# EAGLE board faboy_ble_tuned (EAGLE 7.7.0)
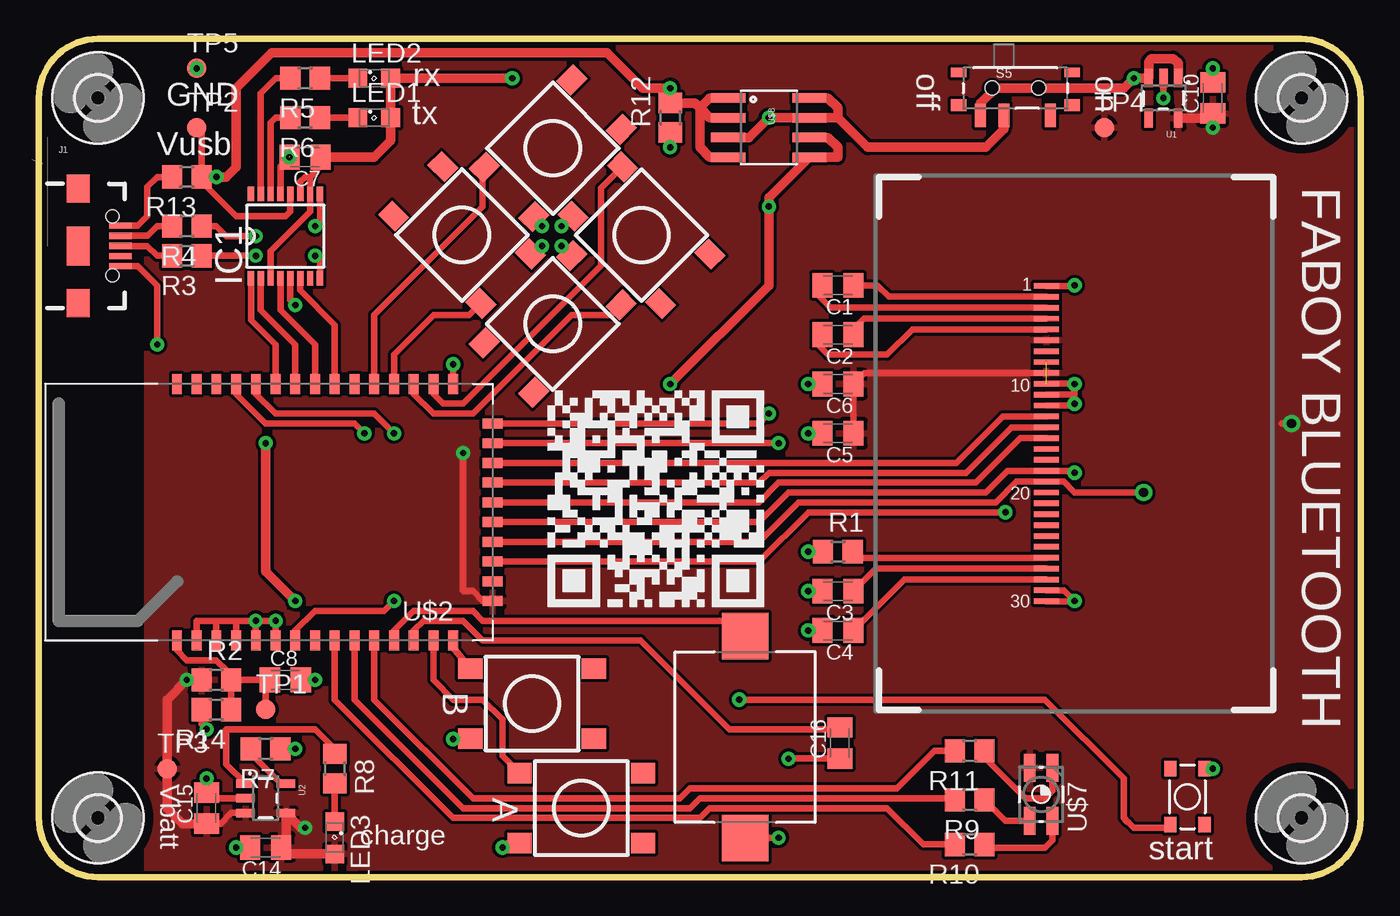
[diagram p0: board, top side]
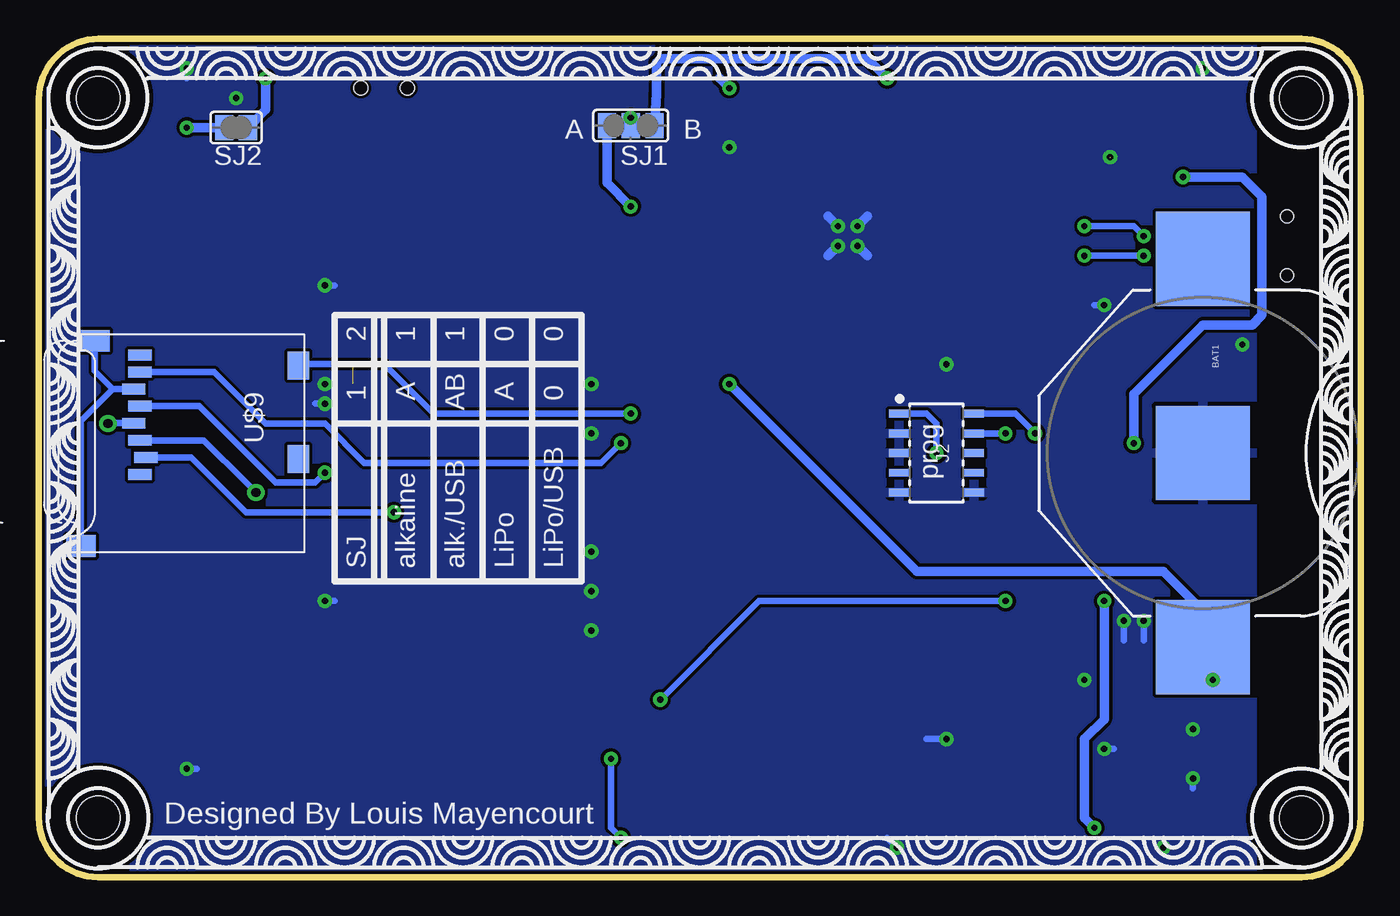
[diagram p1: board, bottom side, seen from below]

Size 85.09 x 53.98 mm. Coordinates in mm from the lower left corner, seen from the top.
Outline: 81.23,53.98 3.81,53.98 arc90 0,50.16 0,3.81 arc90 3.81,0 81.28,0 arc90 85.09,3.81 85.09,50.11 arc90 81.23,53.98
Copper layers (1*16): Top 0.035mm / dielectric 1.5mm / Bottom 0.035mm
Design rules "SparkFun": minimum track width 8mil, minimum drill 20mil, track to track 8mil, track to pad 8mil, pad to pad 8mil, via to via 8mil, smd to smd 8mil, copper to edge 8mil, drill to drill 8mil, minimum pad ring 12mil, minimum via ring 10mil, stop-mask expansion 4mil, vias tented up to drill 20mil, thermal gap 10mil

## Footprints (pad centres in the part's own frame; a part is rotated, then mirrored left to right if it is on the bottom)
BATTCON_20MM = smd 6.07 x 6.07: 1 -12.5,0; 2 0,0; 3 12.5,0
C0805K = smd 1.3 x 1.6: 1 -1,0; 2 1,0
SSOP16 = smd 0.914 x 0.406: 1 -2.718,2.223; 2 -2.718,1.587; 3 -2.718,0.953; 4 -2.718,0.318; 5 -2.718,-0.318; 6 -2.718,-0.953; 7 -2.718,-1.587; 8 -2.718,-2.223; 9 2.718,-2.223; 10 2.718,-1.587; 11 2.718,-0.953; 12 2.718,-0.318; 13 2.718,0.318; 14 2.718,0.953; 15 2.718,1.587; 16 2.718,2.223
USB-B-MICRO-SMD_V03_RED_PASTE = smd 1.45 x 0.4: D+ 2.725,0; D- 2.725,0.65; GND 2.725,-1.3; ID 2.725,-0.65; VBUS 2.725,1.3 | smd 1.5 x 1.8: SHIELD1 0,3.685; SHIELD2 0,-3.685 | smd 1.5 x 2.5: SHIELD3 0,0 | hole 0.85: 2.2,1.9; 2.2,-1.9
SAMTECH_FTSH-105-01 = smd 0.508 x 1.27: 1 -2.54,-2.413; 2 -2.54,2.413; 3 -1.27,-2.413; 4 -1.27,2.413; 5 0,-2.413; 6 0,2.413; 7 1.27,-2.413; 8 1.27,2.413; 9 2.54,-2.413; 10 2.54,2.413
SML0805 = smd 1.2 x 1.2: A 1.05,0; C -1.05,0
R0805 = smd 1.3 x 1.5: 1 -0.95,0; 2 0.95,0
TACTILE_SWITCH_TALL = smd 1.55 x 1.3: A1 -3.975,-2.25; A2 3.975,-2.25; B1 -3.975,2.25; B2 3.975,2.25
SWITCH-SPST-SMD-A = smd 0.7 x 1.5: 1 -2.25,-1.75; 2 -0.75,-1.75; 3 2.25,-1.75 | smd 1 x 0.6: GND1 -3.65,1; GND3 3.65,1 | smd 1 x 0.8: GND2 -3.65,-1.1; GND4 3.65,-1.1 | hole 0.9: -1.5,0; 1.5,0
TACTILE_SWITCH_SMD-3 = smd 1 x 0.8: 1 -1.8,1.1; 2 1.8,1.1; 3 -1.8,-1.1; 4 1.8,-1.1
BUZZER-CMT1102 = smd 3 x 3: 1 -6.5,0; 2 6.5,0
SJ_2 = smd 1.168 x 1.6: 1 -1.524,0; 2 0,0; 3 1.524,0
SJ = smd 1.168 x 1.6: 1 -0.762,0; 2 0.762,0
B1,27 = smd 1.27 x 1.27: TP 0,0
SOT23-5 = smd 0.55 x 1.2: 1 -0.95,-1.3; 2 0,-1.3; 3 0.95,-1.3; 4 0.95,1.3; 5 -0.95,1.3
1X30-0.7MM = smd 0.35 x 1.6: 1 -10.15,0; 2 -9.45,0; 3 -8.75,0; 4 -8.05,0; 5 -7.35,0; 6 -6.65,0; 7 -5.95,0; 8 -5.25,0; 9 -4.55,0; 10 -3.85,0; 11 -3.15,0; 12 -2.45,0; 13 -1.75,0; 14 -1.05,0; 15 -0.35,0; 16 0.35,0; 17 1.05,0; 18 1.75,0; 19 2.45,0; 20 3.15,0; 21 3.85,0; 22 4.55,0; 23 5.25,0; 24 5.95,0; 25 6.65,0; 26 7.35,0; 27 8.05,0; 28 8.75,0; 29 9.45,0; 30 10.15,0
WT51822 = smd 1.27 x 0.635: 1 0,13.97; 2 0,12.7; 3 0,11.43; 4 0,10.16; 5 0,8.89; 6 0,7.62; 7 0,6.35; 8 0,5.08; 9 0,3.81; 10 0,2.54 | smd 0.635 x 1.27: 11 2.54,0; 12 3.81,0; 13 5.08,0; 14 6.35,0; 15 7.62,0; 16 8.89,0; 17 10.16,0; 18 11.43,0; 19 12.7,0; 20 13.97,0; 21 15.24,0; 22 16.51,0; 23 17.78,0; 24 19.05,0; 25 20.32,0; 26 20.32,16.51; 27 19.05,16.51; 28 17.78,16.51; 29 16.51,16.51; 30 15.24,16.51; 31 13.97,16.51; 32 12.7,16.51; 33 11.43,16.51; 34 10.16,16.51; 35 8.89,16.51; 36 7.62,16.51; 37 6.35,16.51; 38 5.08,16.51; 39 3.81,16.51; 40 2.54,16.51
2,8 = hole 2.8: 0,0
P-LCC-4-3 = smd 0.75 x 1.8: 1 0.725,1.7; 2 -0.725,1.7; 3 -0.725,-1.7; 4 0.725,-1.7
SO08 = smd 0.61 x 2.21: 1 -1.905,-2.616; 2 -0.635,-2.616; 3 0.635,-2.616; 4 1.905,-2.616; 5 1.905,2.616; 6 0.635,2.616; 7 -0.635,2.616; 8 -1.905,2.616
MICROSD = smd 0.7 x 1.5: 1 9,-10.64; 2 7.9,-10.24; 3 6.8,-10.64; 4 5.7,-11.04; 5 4.6,-10.64; 6 3.5,-11.04; 7 2.4,-10.64; 8 1.3,-10.64 | smd 1.8 x 1.4: CD1 2,-0.44; CD2 8,-0.44 | smd 1.4 x 1.9: MT1 0.4,-13.54; MT2 13.6,-14.44

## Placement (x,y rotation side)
BAT1  [BATTCON_20MM]  10.16,27.3 270 bottom
C1  1uF  [C0805K]  51.44,38.1 180 top
C2  1uF  [C0805K]  51.44,34.92 180 top
C3  4.7uF / 10v  [C0805K]  51.44,18.41 180 top
C4  2.2uF  [C0805K]  51.44,15.88 180 top
C5  1uF  [C0805K]  51.44,28.57 180 top
C6  1uF  [C0805K]  51.44,31.75 180 top
C7  0.1uF  [C0805K]  17.14,46.35 180 top
C8  22nF  [C0805K]  15.88,12.7 0 top
C10  2.2uF  [C0805K]  75.56,50.16 90 top
C14  4.7uF  [C0805K]  14.61,1.91 180 top
C15  4.7uF  [C0805K]  10.79,4.45 90 top
C16  4.7uF  [C0805K]  51.56,8.64 90 top
IC1  FT230XS  [SSOP16]  15.88,41.27 90 top
J1  USB-MICROBREDUCED_PASTE  [USB-B-MICRO-SMD_V03_RED_PASTE]  2.54,40.64 0 top
J2  CORTEX_DEBUGSMD  [SAMTECH_FTSH-105-01]  27.3,27.3 270 bottom
LED1  [SML0805]  21.59,48.9 0 top
LED2  [SML0805]  21.59,51.44 0 top
LED3  [SML0805]  19.05,2.54 270 top
R1  390k  [R0805]  51.44,20.95 0 top
R2  10M  [R0805]  11.43,12.7 0 top
R3  22  [R0805]  9.53,40.01 180 top
R4  22  [R0805]  9.53,41.91 180 top
R5  820  [R0805]  17.14,51.44 180 top
R6  820  [R0805]  17.14,48.9 180 top
R7  390k  [R0805]  14.61,8.26 180 top
R8  470  [R0805]  19.05,6.99 270 top
R9  820  [R0805]  59.92,4.98 180 top
R10  820  [R0805]  59.92,2.11 180 top
R11  820  [R0805]  59.92,8.13 180 top
R12  10k  [R0805]  40.64,48.9 90 top
R13  ferrite  [R0805]  9.53,45.09 180 top
R14  2.2M  [R0805]  11.43,10.79 180 top
S1  SWITCH-MOMENTARY-2SMD-4  [TACTILE_SWITCH_TALL]  38.79,41.33 135 top
S2  SWITCH-MOMENTARY-2SMD-4  [TACTILE_SWITCH_TALL]  33.08,35.62 45 top
S3  SWITCH-MOMENTARY-2SMD-4  [TACTILE_SWITCH_TALL]  33.09,46.93 225 top
S4  SWITCH-MOMENTARY-2SMD-4  [TACTILE_SWITCH_TALL]  27.24,41.34 315 top
S5  [SWITCH-SPST-SMD-A]  62.87,50.8 0 top
S6  SWITCH-MOMENTARY-2SMD-4  [TACTILE_SWITCH_TALL]  34.92,4.45 180 top
S7  SWITCH-MOMENTARY-2SMD-4  [TACTILE_SWITCH_TALL]  31.75,11.18 180 top
S8  SWITCH-MOMENTARY-2SMD-3  [TACTILE_SWITCH_SMD-3]  73.94,5.18 270 top
SG1  BUZZERSMD3  [BUZZER-CMT1102]  45.47,9.02 270 top
SJ1  conf_1  [SJ_2]  46.99,48.39 180 bottom
SJ2  conf_2  [SJ]  72.39,48.26 180 bottom
TP1  TPB1,27  [B1,27]  14.61,10.79 0 top
TP2  TPB1,27  [B1,27]  10.16,48.26 0 top
TP3  TPB1,27  [B1,27]  8.26,6.99 0 top
TP4  TPB1,27  [B1,27]  68.58,48.26 0 top
TP5  TPB1,27  [B1,27]  10.16,52.07 0 top
U1  3.3V/150mA  [SOT23-5]  72.39,50.16 180 top
U2  MCP73831  [SOT23-5]  14.61,5.08 270 top
U$1  UG-2864HSWEG01  [1X30-0.7MM]  64.87,27.91 270 top
U$2  WT51822-02  [WT51822]  29.21,31.75 180 top
U$3  [2,8]  81.28,50.16 270 top
U$4  [2,8]  81.28,3.81 270 top
U$5  gnd  [2,8]  3.81,50.16 270 top
U$6  [2,8]  3.81,3.81 270 top
U$7  LED-RGB-P-LCC-4  [P-LCC-4-3]  64.52,5.33 0 top
U$8  SI4833BDY  [SO08]  46.99,48.26 270 top
U$9  MICROSD  [MICROSD]  67.94,34.92 270 bottom

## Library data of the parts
BAT1 S8 SG1 = SparkFun-Electromechanical
C1-C8 C10 C14-C16 R1-R14 = resistor
IC1 = ftdichip
J1 = SparkFun-Connectors; PROD_ID: CONN-11752
J2 = SparkFun-Connectors
LED1-LED3 = led
S1-S4 S6 S7 = SparkFun-Electromechanical; PROD_ID: SWCH-11966
S5 = SparkFun-Electromechanical; PROD_ID: SWCH-10651
SJ1 SJ2 = jumper
TP1-TP5 = testpad
U1 = SparkFun-PowerIC; PROD_ID: VREG-00822
U2 = SparkFun-PowerIC; PROD_ID: IC-09995
U$1 U$9 = adafruit
U$2 = Wireless_Tag
U$3-U$6 = holes
U$7 = SparkFun-LED
U$8 = SparkFun-DiscreteSemi

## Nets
3V3: C7.1 IC1.3 IC1.10 IC1.11 LED1.A LED2.A SJ1.1
A: S7.A2 U$2.40
B: S6.A2 U$2.39
BLUE: R9.2 U$2.35
CS_OLED: U$1.13 U$2.8
CS_SD: U$2.3 U$9.2
CTS: IC1.6 U$2.17
D+: IC1.8 R3.1
D-: IC1.9 R4.1
DC: U$1.15 U$2.6
DOWN: S4.A2 U$2.14
GND: BAT1.2 C3.2 C4.2 C5.2 C6.2 C7.2 C8.2 C10.2 C14.2 C15.2 IC1.5 IC1.13 J1.GND J2.3 J2.5 J2.9 J2.10 R1.1 R7.1 R12.1 R14.2 S1.B2 S2.B2 S3.B2 S4.B2 S6.B2 S7.B2 S8.1 TP5.TP U1.2 U2.2 U$1.1 U$1.8 U$1.10 U$1.11 U$1.12 U$1.29 U$1.30 U$2.11 U$2.27 U$2.28 U$2.29 U$2.30 U$2.31
GREEN: R10.2 U$2.34
LED_RX: IC1.15 R5.2
LED_TX: IC1.14 R6.2
LEFT: S3.A2 U$2.15
MES_BAT: C8.1 R2.2 R14.1 TP1.TP U$2.26
MISO: U$2.9 U$9.7
MOSI: U$1.19 U$2.4 U$9.3
N$1: C1.1 U$1.2
N$2: C1.2 U$1.3
N$3: C2.1 U$1.4
N$4: C2.2 U$1.5
N$5: R1.2 U$1.26
N$6: R11.1 U$7.1
N$7: C3.1 U$1.27
N$8: C4.1 U$1.28
N$9: S5.1 SJ2.1 U1.1 U1.3
N$10: C16.2 U$2.38
N$11: C16.1 SG1.2
N$12: J1.D+ R3.2
N$13: J1.D- R4.2
N$17: R8.1 U2.1
N$18: LED3.C R8.2
N$19: R7.2 U2.5
N$21: SG1.1 U$2.37
N$22: R10.1 U$7.4
N$23: LED2.C R5.1
N$24: R9.1 U$7.3
N$25: LED1.C R6.1
N$28: S5.2 SJ1.2 U$8.3 U$8.7 U$8.8
OLED_RST: U$1.14 U$2.7
RED: R11.2 U$2.36
RIGHT: S2.A2 U$2.13
RST: S8.4 U$2.32
RTS: IC1.2 U$2.19
RX: IC1.4 U$2.18
SCLK: U$1.18 U$2.5 U$9.5
SD_DETECT: U$2.10 U$9.CD1
SWDCLK: J2.4 U$2.21
SWDIO: J2.2 U$2.22
TX: IC1.1 U$2.20
UP: S1.A2 U$2.12
VBAT: BAT1.3 C15.1 R2.1 SJ1.3 TP3.TP U2.3 U$8.5 U$8.6
VBUS: J1.VBUS R13.2
VCC: C5.1 C6.1 C10.1 J2.1 SJ2.2 TP4.TP U1.5 U$1.6 U$1.9 U$2.1 U$7.2 U$9.4
VIN: C14.1 IC1.12 LED3.A R12.2 R13.1 TP2.TP U2.4 U$8.1 U$8.2 U$8.4
VSS: U$9.6 U$9.MT1 U$9.MT2

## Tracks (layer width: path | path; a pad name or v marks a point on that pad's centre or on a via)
3V3  (via drill 0.4)
  Top 0.406: IC1.11 16.83,44.77 17.14,45.09 17.46,45.09 | 17.46,45.09 IC1.10 17.46,42.86 14.92,40.32 IC1.3 | C7.1 18.14,45.77 17.46,45.09
  Top 0.61: C7.1 21.59,46.35 22.64,47.41 LED1.A LED2.A v30.48,51.44
  Bottom 0.61: v30.48,51.44 31.75,52.7 45.09,52.7 45.34,52.45 45.34,50.42 SJ1.1
A
  Top 0.406: S7.A2 26.67,14.79 U$2.40
B
  Top 0.406: S6.A2 29.84,7.8 29.84,10.16 28.57,11.43 26.67,11.43 25.4,12.7 U$2.39
BLUE
  Top 0.406: U$2.35 20.32,11.43 27.3,4.45 41.91,4.45 42.55,5.08 58.87,5.08 R9.2
CS_OLED
  Top 0.406: U$1.13 62.05,29.66 59.05,26.67 U$2.8
CS_SD  (via drill 0.4)
  Top 0.406: U$2.3 46.35,20.32 49.53,23.5 v62.23,23.5
  Bottom 0.406: v62.23,23.5 71.75,23.5 75.28,27.02 U$9.2
CTS
  Top 0.406: IC1.6 16.83,37.78 19.05,35.56 U$2.17
D+  (via drill 0.4)
  Top 0.406: R3.1 v13.97,40.01 | v17.78,40.01 18.1,39.69 IC1.8
  Bottom 0.406: v13.97,40.01 v17.78,40.01
D-  (via drill 0.4)
  Top 0.406: v13.97,41.27 12.06,41.27 11.43,41.91 R4.1 | v17.78,41.91 18.1,42.23 IC1.9
  Bottom 0.406: v13.97,41.27 14.61,41.91 v17.78,41.91
DC
  Top 0.406: U$1.15 63.19,28.27 60.33,25.4 47.62,25.4 46.35,24.13 U$2.6
DOWN
  Top 0.406: U$2.14 22.86,33.66 25.4,36.2 27.71,36.2 S4.A2
GND  (via drill 0.4)  (2 unrouted)
  Top 0.406: IC1.13 15.56,45.77 16.13,46.34 v16.13,46.35 | C15.2 arc90 11.16,5.08 U2.2 11.43,5.08 10.79,5.71 v10.79,6.35 | C4.2 v49.53,15.88 | C3.2 v49.53,18.41 | R1.1 v49.53,20.95 | C5.2 v49.53,28.57 | U1.2 v72.39,50.16 | U$2.11 v26.67,33.02 | J1.GND 6.38,39.34 7.62,38.1 v7.62,34.29 | C14.2 v12.7,1.91 | U$1.29 65.99,18.46 v66.67,17.78 66.66,17.77 U$1.30 | S8.1 v75.56,6.98 v75.56,6.99 | U$1.10 66.66,31.77 v66.67,31.75 66.67,31.11 66.62,31.07 | U$1.12 66.56,30.36 v66.67,30.48 66.67,31.02 66.62,31.07 | U$1.11 66.62,31.07 | C10.2 v75.56,52.07 | C6.2 v49.53,31.75 | S6.B2 30.14,2.19 v29.84,1.91 | S7.B2 26.71,8.93 v26.67,8.89 | R7.1 v16.51,8.26 | R14.2 10.48,9.84 v10.79,9.53 | C8.2 v17.78,12.7 | U$2.31 v15.24,16.51 12.7,16.51 U$2.29 | U$2.30 v13.97,16.51 11.43,16.51 | U$2.27 10.16,16.51 11.43,16.51 | U$2.28 11.43,16.51 | IC1.5 16.19,37.15 v16.51,36.83 | U$1.1 66.64,38.06 v66.67,38.1
  Top 0.61: R12.1 v40.64,46.99 | S4.B2 31.87,40.12 v32.38,40.64 | S3.B2 31.87,42.43 v32.38,41.91 | S1.B2 34.3,42.55 v33.66,41.91 | S2.B2 34.27,40.02 v33.66,40.64
  Bottom 0.406: v66.67,17.78 66.04,17.78 | v75.56,6.99 74.93,6.99 | v66.67,31.75 66.04,31.75 | v66.67,30.48 67.31,30.48 | v75.56,52.07 75.56,51.44 | v49.53,31.75 50.16,31.75 | v29.84,1.91 30.48,2.54 | v26.67,8.89 27.94,8.89 | v16.51,8.26 15.88,8.26 | v10.79,6.35 10.79,5.71 | v15.24,16.51 U$2.31 | v13.97,16.51 U$2.30 | v16.51,36.83 17.14,36.83 | v66.67,38.1 66.04,38.1
  Bottom 0.61: v32.38,40.64 31.75,40.01 | v32.38,41.91 31.75,42.55 | v33.66,41.91 34.29,42.55 | v33.66,40.64 34.29,40.01
  other vias: 10.16,52.07
  pour Bottom: 6.99,53.98 85.09,53.98 85.09,0 6.99,0
GREEN
  Top 0.406: U$2.34 19.05,11.43 26.67,3.81 42.55,3.81 43.18,4.45 54.61,4.45 56.95,2.11 R10.2
LED_RX
  Top 0.406: IC1.15 14.29,50.48 15.24,51.44 R5.2
LED_TX
  Top 0.406: IC1.14 14.92,48.58 15.24,48.9 R6.2
LEFT
  Top 0.406: U$2.15 21.59,36.2 28.57,43.18 28.57,45.6 S3.A2
MES_BAT
  Top 0.406: U$2.26 8.89,14.61 9.53,13.97 11.43,13.97 12.06,13.34 12.06,13.02 R2.2 | R14.1 R2.2 | R2.2 C8.1 14.61,12.43 TP1.TP
MISO  (via drill 0.4)
  Top 0.406: U$2.9 v47.62,27.94
  Bottom 0.406: v47.62,27.94 48.9,26.67 64.14,26.67 66.67,29.21 70.48,29.21 73.8,32.52 U$9.7
MOSI  (via drill 0.6)
  Top 0.406: U$2.4 46.35,21.59 48.9,24.13 61.59,24.13 62.93,25.46 U$1.19 65.97,25.46 66.67,24.77 v71.12,24.77
  Bottom 0.406: U$9.3 74.48,28.12 71.75,25.4 v71.12,24.77
N$1
  Top 0.406: U$1.2 54.71,37.37 53.98,38.1 C1.1
N$2
  Top 0.406: U$1.3 50.97,36.66 50.16,37.47 50.16,37.83 C1.2
N$3
  Top 0.406: U$1.4 53.11,35.97 52.7,35.56 52.7,35.2 C2.1
N$4
  Top 0.406: U$1.5 56.22,35.27 54.61,33.66 50.8,33.66 50.16,34.29 50.16,34.66 C2.2 50.8,34.56
N$5
  Top 0.406: U$1.26 52.77,20.57 R1.2
N$6
  Top 0.406: U$7.1 65.24,5.55 64.77,5.08 63.5,5.08 60.96,7.62 60.96,8.04 R11.1
N$7
  Top 0.406: U$1.27 53.88,19.86 C3.1
N$8
  Top 0.406: U$1.28 55.73,19.16 C4.1
N$9  (via drill 0.4)
  Top 0.61: S5.1 60.62,49.82 61.59,50.8 69.85,50.8 v70.48,51.44 71.41,51.44 U1.3 71.44,52.52 71.63,52.7 73.03,52.7 73.34,52.39 U1.1
  Bottom 0.61: v70.48,51.44 70.48,49.4 SJ2.1
N$10
  Top 0.406: U$2.38 24.13,15.88 24.77,16.51 27.3,16.51 28.57,15.24 38.73,15.24 44.45,9.53 51.45,9.53 C16.2
N$11  (via drill 0.4)
  Top 0.406: C16.1 48.28,7.64 v48.26,7.62 | v47.62,2.54 45.49,2.54 SG1.2
  Bottom 0.406: v48.26,7.62 48.26,3.17 v47.62,2.54
N$12
  Top 0.406: J1.D+ 6.99,40.64 7.62,40.01 R3.2
N$13
  Top 0.406: J1.D- 7,41.29 7.62,41.91 R4.2
N$17
  Top 0.406: U2.1 12.06,7.27 12.06,9.53 17.78,9.53 19.05,8.26 R8.1
N$18
  Top 0.406: R8.2 LED3.C
N$19
  Top 0.406: U2.5 15.56,6.03 13.65,7.93 R7.2
N$21
  Top 0.406: U$2.37 22.86,15.88 24.13,17.14 27.94,17.14 28.57,16.51 44.47,16.51 SG1.1
N$22
  Top 0.406: U$7.4 65.24,2.38 64.77,1.91 61.07,1.91 R10.1
N$23
  Top 0.406: R5.1 LED2.C
N$24
  Top 0.406: U$7.3 62.21,3.63 R9.1
N$25
  Top 0.406: R6.1 LED1.C
N$28  (via drill 0.4)
  Top 0.61: S5.2 62.12,48.15 60.96,46.99 53.34,46.99 51.44,48.9 | 51.44,48.9 U$8.7 v46.99,48.9 45.72,47.62 U$8.3 | U$8.8 50.8,50.16 51.44,49.53 51.44,48.9
  Bottom 0.61: SJ1.2 v46.99,48.9
OLED_RST
  Top 0.406: U$1.14 62.62,28.96 59.69,26.04 46.99,26.04 46.35,25.4 U$2.7
RED
  Top 0.406: R11.2 57.66,8.13 55.24,5.71 41.91,5.71 41.27,5.08 27.94,5.08 21.59,11.43 U$2.36
RIGHT
  Top 0.406: U$2.13 24.13,31.11 25.4,29.84 27.94,29.84 34.29,36.2 36.84,36.2 S2.A2
RST  (via drill 0.4)
  Top 0.406: S8.4 72.63,3.17 70.48,3.17 70.17,3.49 70.05,3.61 69.85,3.81 69.85,6.35 64.77,11.43 v45.09,11.43 | U$2.32 16.51,15.88 17.78,17.14 22.23,17.14 v22.86,17.78
  Bottom 0.406: v22.86,17.78 38.73,17.78 v45.09,11.43
RTS
  Top 0.406: IC1.2 14.29,36.51 16.51,34.29 U$2.19
RX
  Top 0.406: IC1.4 15.56,36.51 17.78,34.29 U$2.18
SCLK  (via drill 0.4)
  Top 0.406: U$2.5 46.35,22.86 48.26,24.77 60.96,24.77 62.36,26.16 U$1.18 66.55,26.16 v66.67,26.04
  Bottom 0.406: v66.67,26.04 67.31,25.4 69.85,25.4 74.78,30.32 U$9.5
SD_DETECT  (via drill 0.4)
  Top 0.406: U$2.10 46.35,29.21 v46.99,29.84
  Bottom 0.406: v46.99,29.84 59.69,29.84 62.87,33.02 68.29,33.02 U$9.CD1
SWDCLK  (via drill 0.4)
  Top 0.406: U$2.21 13.97,31.11 15.24,29.84 21.59,29.84 v22.86,28.57
  Bottom 0.406: v22.86,28.57 J2.4
SWDIO  (via drill 0.4)
  Top 0.406: U$2.22 12.7,31.11 14.61,29.21 20.32,29.21 v20.95,28.57
  Bottom 0.406: v20.95,28.57 22.23,29.84 J2.2
TX
  Top 0.406: IC1.1 13.65,35.88 15.24,34.29 U$2.20
UP
  Top 0.406: U$2.12 25.4,31.11 26.04,30.48 27.3,30.48 36.2,39.37 36.2,44.36 S1.A2
VBAT  (via drill 0.4)
  Top 0.406: C15.1 11.7,3.44 12.38,4.13 U2.3
  Top 0.61: C15.1 9.26,3.44 8.26,4.45 TP3.TP 8.26,11.43 v9.53,12.7 R2.1 | U$8.6 50.8,47.62 51.44,46.99 51.44,46.35 U$8.5 46.99,43.74 v46.99,43.18 46.99,38.1 v40.64,31.75
  Bottom 0.61: v9.53,12.7 10.16,13.34 BAT1.3 10.16,17.14 12.7,19.68 28.57,19.68 v40.64,31.75 | v46.99,43.18 48.51,44.7 SJ1.3
  pour Top: 13.34,0 6.99,0 6.99,13.97 13.34,13.97
VBUS
  Top 0.406: J1.VBUS 6.38,41.94 6.99,42.55 6.99,44.45 7.62,45.09 R13.2
VCC  (via drill 0.4, 0.6)
  Top 0.406: U$1.9 53.15,32.47 C6.1 C5.1 | v27.3,27.3 27.3,18.41 27.94,18.41 28.57,17.78 U$2.1 | v80.64,29.21 80.01,29.21
  Top 0.61: U1.5 75.27,48.87 C10.1 v75.56,48.26
  Bottom 0.406: U$9.4 80.63,29.23 v80.64,29.21 | v27.3,27.3 27.3,29.21 27.94,29.84 J2.1
  Bottom 0.61: v75.56,48.26 SJ2.2
  pour Top: 6.99,53.98 84.45,53.98 84.45,0.64 6.99,0.64
VIN  (via drill 0.4)
  Top 0.406: IC1.12 16.19,42.86 15.88,42.55 12.7,42.55 10.47,44.77 R13.1 10.47,47.95 TP2.TP
  Top 0.61: LED3.A 15.61,1.49 C14.1 15.9,1.91 U2.4 16.86,3.17 v17.14,3.17 | v11.43,45.09 R13.1 12.06,45.09 12.7,45.72 12.7,50.8 14.99,53.09 36.58,53.09 38.86,50.8 v40.64,50.8 R12.2 42.23,49.84 42.55,49.53 | v14.61,27.94 14.61,19.68 v16.51,17.78 | U$8.1 43.18,50.16 42.55,49.53 | 42.55,49.53 43.18,48.9 U$8.2 | U$8.4 43.18,46.35 42.55,46.99 42.55,49.53
  Bottom 0.61: v11.43,45.09 7.62,45.09 6.35,43.81 6.35,36.2 6.99,35.56 10.16,35.56 14.61,31.11 v14.61,27.94 | v16.51,17.78 16.51,10.16 17.78,8.89 17.78,3.81 v17.14,3.17 | 41.27,51.44 v40.64,50.8
  pour Top: 14.61,0 20.32,0 20.32,4.45 14.61,4.45
VSS
  Bottom 0.406: U$9.MT1 81.48,32.59 80.32,31.43 | 80.32,31.43 U$9.6 | U$9.MT2 82.39,29.36 80.32,31.43

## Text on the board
tPlace: off | on | rx | GND | tx | Vusb | FABOY BLUETOOTH | B | Vbatt | A | charge | start
bPlace: B | A | 0 | 0 | 1 | 1 | 2 | 0 | A | A | 1 | AB | prog | LiPo/USB | LiPo | alk./USB | alkaline | SJ | Designed By Louis Mayencourt

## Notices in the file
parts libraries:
SparkFun-Electromechanical: Licensing: Creative Commons ShareAlike 4.0 International - https://creativecommons.org/licenses/by-sa/4.0
